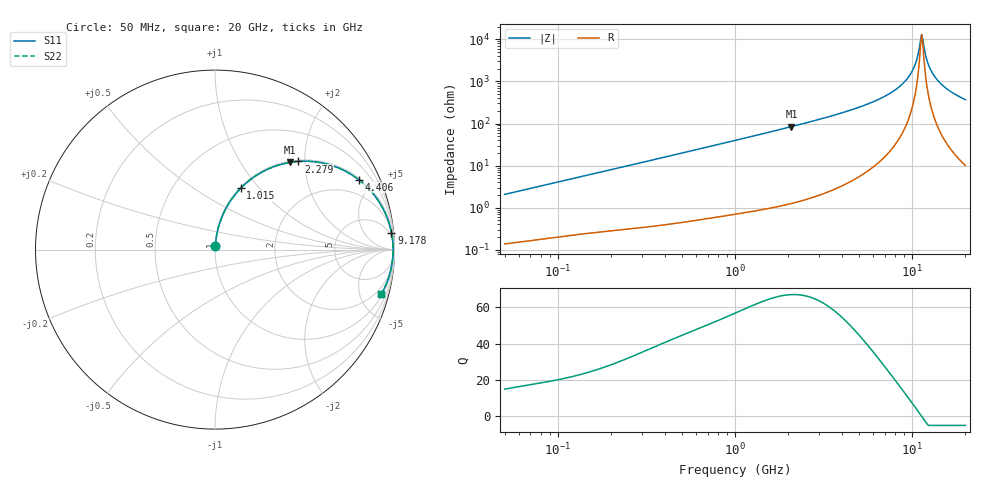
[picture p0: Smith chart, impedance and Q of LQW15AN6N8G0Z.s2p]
!Murata Part Number: LQW15AN6N8G0Z
!These Parameters are Measured in Series Mode Connection
!  o--[Z]--o
!Port1  Port2
!  o-------o
!Freq. Start=50[MHz] Stop=20[GHz], 401[Steps]
# Hz S RI R 50
!Freq.(Hz) S11(Real) S11(Imag) S21(Real) S21(Imag) S12(Real) S12(Imag) S22(Real) S22(Imag)
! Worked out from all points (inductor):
!   401 points, 50 MHz to 20 GHz, reference 50 ohm
!   read as one part in series: L = 6.54 nH near 51.52 MHz
!   highest Q = 67 at 2.083 GHz (marker M1), where L = 6.44 nH
!   self-resonance near 11.32 GHz
!   S11 on the Smith chart (normalised r, x): 50 MHz: 1.00, +0.04; 1.015 GHz: 1.01, +0.80; 2.279 GHz: 1.03, +1.86; 4.406 GHz: 1.08, +4.05; 9.178 GHz: 3, +21; 20 GHz: 1.20, -7.39
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5e7  0.0018 0.0206  0.9982 -0.0206  0.9982 -0.0206  0.0018 0.0206
1.364002e8  0.00536 0.0546  0.9946 -0.0546  0.9946 -0.0546  0.00536 0.0546
3.721004e8  0.0249 0.1436  0.9751 -0.1436  0.9751 -0.1436  0.0249 0.1436
1e9  0.14 0.3382  0.86 -0.3382  0.86 -0.3382  0.14 0.3382
1.015091e9  0.1435 0.3419  0.8565 -0.3419  0.8565 -0.3419  0.1435 0.3419
2.083303e9  0.4171 0.4857  0.5829 -0.4857  0.5829 -0.4857  0.4171 0.4857
2.279204e9  0.4639 0.4913  0.5361 -0.4913  0.5361 -0.4913  0.4639 0.4913
2.728004e9  0.5608 0.4887  0.4392 -0.4887  0.4392 -0.4887  0.5608 0.4887
4.405649e9  0.7996 0.3905  0.2004 -0.3905  0.2004 -0.3905  0.7996 0.3905
5.944466e9  0.9047 0.2801  0.0953 -0.2801  0.0953 -0.2801  0.9047 0.2801
7.442007e9  0.9559 0.1856  0.0441 -0.1856  0.0441 -0.1856  0.9559 0.1856
9.178299e9  0.9833 0.0938  0.0167 -0.0938  0.0167 -0.0938  0.9833 0.0938
1.019291e10  0.9901 0.0473  0.00992 -0.0473  0.00992 -0.0473  0.9901 0.0473
1.066139e10  0.9916 0.0274  0.00837 -0.0274  0.00837 -0.0274  0.9916 0.0274
1.115139e10  0.9924 0.00738  0.00764 -0.00738  0.00764 -0.00738  0.9924 0.00738
1.131968e10  0.9924 0.000717  0.00757 -0.000717  0.00757 -0.000717  0.9924 0.000717
1.166392e10  0.9923 -0.0126  0.00771 0.0126  0.00771 0.0126  0.9923 -0.0126
1.201863e10  0.9918 -0.0259  0.00821 0.0259  0.00821 0.0259  0.9918 -0.0259
1.238412e10  0.9909 -0.0393  0.00906 0.0393  0.00906 0.0393  0.9909 -0.0393
1.354865e10  0.9862 -0.0792  0.0138 0.0792  0.0138 0.0792  0.9862 -0.0792
1.597544e10  0.9688 -0.1519  0.0312 0.1519  0.0312 0.1519  0.9688 -0.1519
2e10  0.926 -0.2485  0.074 0.2485  0.074 0.2485  0.926 -0.2485
